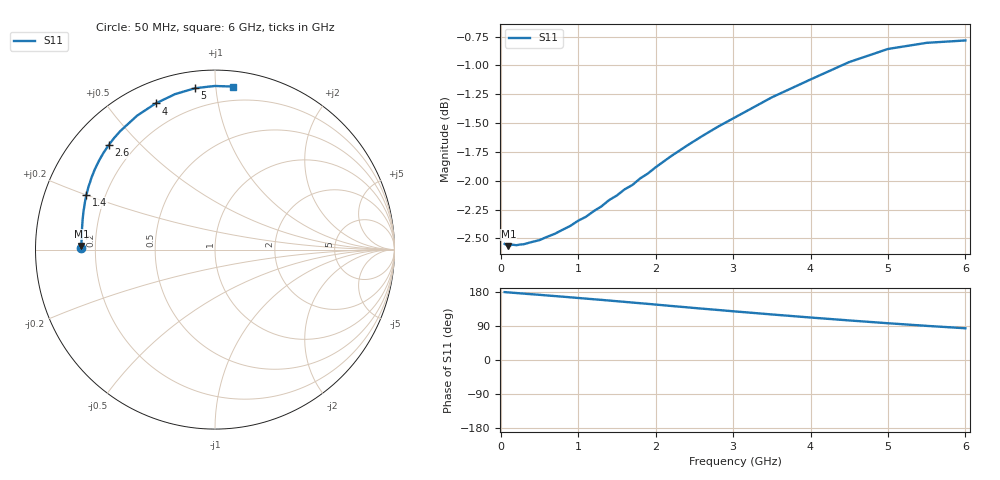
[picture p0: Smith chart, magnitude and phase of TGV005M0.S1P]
! SIEMENS Discrete & RF Semiconductors
! BAT64
! Si Schottky Diode in SOT23
! IF = 5 mA
! S-Parameters:  February  1997
# GHz  S  MA  R  50
!  f  S11
! GHz  MAG  ANG
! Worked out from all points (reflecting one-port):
!   34 points, 50 MHz to 6 GHz, reference 50 ohm
!   lowest |S11| = -2.6 dB at 100 MHz (marker M1), VSWR 6.82, Z = 7.34 + j0.683 ohm
!   phase of S11 starts at 179 deg and turns -95 deg over the sweep
!   S11 on the Smith chart (normalised r, x): 50 MHz: 0.15, +0.01; 1.4 GHz: 0.13, +0.20; 2.6 GHz: 0.11, +0.41; 4 GHz: 0.09, +0.67; 5 GHz: 0.09, +0.88; 6 GHz: 0.10, +1.11
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0.05  0.7458 179.2
0.1  0.7441 178.4
0.15  0.7452 177.5
0.2  0.7448 176.8
0.25  0.7453 175.9
0.4  0.7472 173.5
0.5  0.7486 172.0
0.6  0.7511 170.3
0.8  0.7564 167.1
1  0.7633 163.7
1.2  0.7706 160.3
1.3  0.7742 158.7
1.4  0.7792 156.9
1.6  0.7875 153.4
1.7  0.791 151.6
1.8  0.7962 149.9
2  0.8051 146.3
2.2  0.8141 142.6
2.4  0.8225 139.1
2.6  0.8305 135.5
2.8  0.8382 132.1
3  0.8453 128.6
3.5  0.8633 120.2
4  0.8789 112.1
4.5  0.8943 104.4
5  0.9061 97.0
5.5  0.9116 90.1
6  0.9138 83.7
